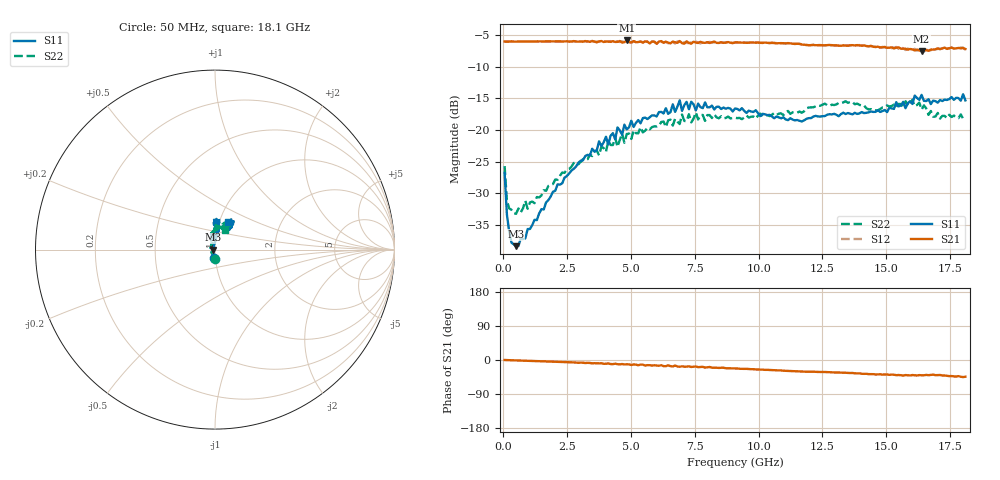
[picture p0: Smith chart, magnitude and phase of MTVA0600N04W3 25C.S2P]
! Network Analyzer HP8720D.06.14 Serial No. US36140669
!  8 Jul 2005  11:27:33
! Frequency  S11  S21  S12  S22
# HZ  S  DB R 50
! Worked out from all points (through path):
!   201 points, 50 MHz to 18.1 GHz, reference 50 ohm
!   highest |S21| = -5.89 dB at 4.833 GHz (marker M1); lowest = -7.6 dB at 16.39 GHz (marker M2)
!   group delay of S21, straight-line fit = 7 ps
!   lowest |S11| = -38.3 dB at 501.2 MHz (marker M3), VSWR 1.02, Z = 48.8 + j0.00331 ohm
!   |S11| at or under -10 dB: start of sweep to end of sweep
!   |S22| runs from -33.2 to -15.2 dB; largest |S21 - S12| = 0.02
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5e7  -26.74 -97.7  -6.04 -0.0  -6.05 0.0  -25.70 -89.7
1.4025e8  -33.35 -115.2  -6.09 -0.2  -6.07 -0.2  -31.18 -133.1
2.305e8  -36.07 -133.8  -6.07 -0.3  -6.06 -0.4  -32.38 -152.7
5.0125e8  -38.32 179.8  -6.07 -1.1  -6.07 -1.1  -33.20 176.3
2.12575e9  -28.57 92.8  -6.03 -5.1  -6.04 -5.0  -27.85 115.1
3.1185e9  -24.79 89.1  -6.06 -7.1  -6.08 -7.5  -24.59 111.9
4.021e9  -21.07 86.1  -6.04 -9.9  -6.11 -9.2  -23.46 102.8
4.382e9  -21.48 83.6  -6.12 -9.7  -6.07 -11.0  -21.22 102.8
4.47225e9  -19.60 79.8  -6.11 -11.1  -6.03 -10.1  -22.67 105.4
4.83325e9  -19.91 88.6  -5.89 -11.3  -6.03 -12.4  -20.64 92.9
6.09675e9  -17.18 83.0  -6.06 -15.0  -6.00 -14.9  -19.34 91.3
6.7285e9  -17.14 89.4  -6.18 -14.8  -6.37 -15.8  -18.24 85.7
6.909e9  -15.32 87.5  -5.98 -18.0  -6.14 -16.7  -19.07 83.7
6.99925e9  -16.99 87.0  -6.31 -16.5  -6.37 -18.2  -17.56 85.3
7.17975e9  -15.57 91.9  -6.02 -17.4  -6.27 -16.8  -18.61 80.4
7.54075e9  -16.91 83.8  -6.22 -17.0  -6.06 -19.2  -17.24 88.8
9.075e9  -16.62 90.7  -6.20 -22.2  -6.18 -22.3  -18.08 78.3
1.21435e10  -17.89 77.6  -6.59 -30.8  -6.56 -30.9  -16.42 71.3
1.512175e10  -16.49 55.3  -7.03 -39.2  -6.89 -38.7  -16.29 69.9
1.602425e10  -15.90 59.8  -7.29 -39.7  -7.42 -41.7  -15.23 63.0
1.638525e10  -14.47 56.5  -7.59 -40.4  -7.39 -39.6  -16.79 61.5
1.81e10  -15.33 64.4  -7.23 -44.0  -7.36 -44.9  -18.13 64.2
